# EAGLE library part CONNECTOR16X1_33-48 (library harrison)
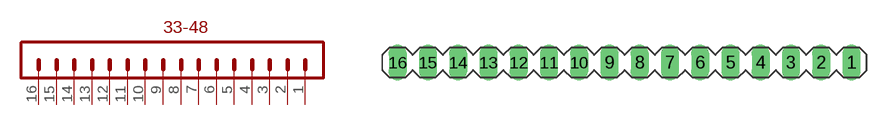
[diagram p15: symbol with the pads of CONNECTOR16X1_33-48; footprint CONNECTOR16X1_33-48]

Designator prefix -

## CONNECTOR16X1_33-48  [CONNECTOR16X1_33-48]
1  P$1  pas
2  P$2  pas
3  P$3  pas
4  P$4  pas
5  P$5  pas
6  P$6  pas
7  P$7  pas
8  P$8  pas
9  P$9  pas
10  P$10  pas
11  P$11  pas
12  P$12  pas
13  P$13  pas
14  P$14  pas
15  P$15  pas
16  P$16  pas

## Footprint CONNECTOR16X1_33-48 (pad centres in mm)
drill 1.016 long: 1 17.78,0.635; 2 15.24,0.635; 3 12.7,0.635; 4 10.16,0.635; 5 7.62,0.635; 6 5.08,0.635; 7 2.54,0.635; 8 0,0.635; 9 -2.54,0.635; 10 -5.08,0.635; 11 -7.62,0.635; 12 -10.16,0.635; 13 -12.7,0.635; 14 -15.24,0.635; 15 -17.78,0.635; 16 -20.32,0.635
